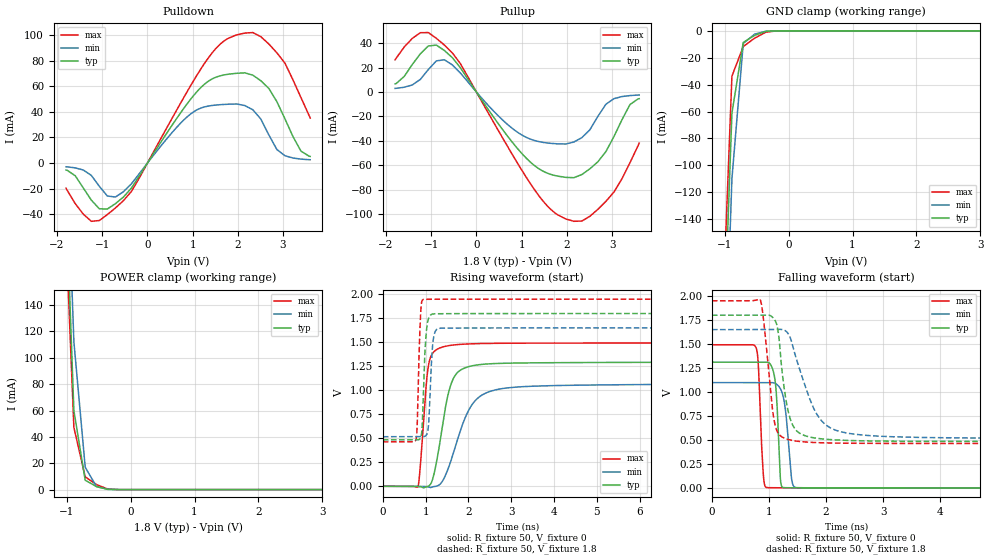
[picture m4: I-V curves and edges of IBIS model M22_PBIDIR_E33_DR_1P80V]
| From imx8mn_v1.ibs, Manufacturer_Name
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[Model] M22_PBIDIR_E33_DR_1P80V
Model_type I/O
Vinl  =  0.54
Vinh  =  1.26
Vmeas =  0.9
| Capacitance   typ   min   max
C_comp   8.99140471561e-13   8.21462742958e-13   9.40633374847e-13
| Variables   typ   min   max
[GND Clamp Reference]   0   0   0
[POWER Clamp Reference]   1.8   1.65   1.95
[Pulldown Reference]   0   0   0
[Pullup Reference]   1.8   1.65   1.95
[Temperature Range]   25   125   -40
[Voltage Range]   1.8   1.65   1.95
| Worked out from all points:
|   slope of the pulldown table from 0 to 0.27 V, typ, clamps not added: 18.2 ohm
|   slope of the pullup table from 0 to 0.27 V, typ, clamps not added: 18.3 ohm
|   GND clamp passes 1 mA (typ) near -0.39 V on its own axis
|   POWER clamp passes 1 mA (typ) near -0.43 V on its own axis
|   falling waveform, R_fixture 50, V_fixture 0: 20-80 % time 64.8ps typ, 101ps min, 63.2ps max; typ from 1.31 V to 0 V
|   falling waveform, R_fixture 50, V_fixture 1.8: 20-80 % time 178ps typ, 425ps min, 151ps max; typ from 1.8 V to 0.484 V
|   rising waveform, R_fixture 50, V_fixture 0: 20-80 % time 321ps typ, 562ps min, 154ps max; typ from 0 V to 1.3 V
|   rising waveform, R_fixture 50, V_fixture 1.8: 20-80 % time 72.2ps typ, 72.2ps min, 56.6ps max; typ from 0.484 V to 1.8 V
[GND Clamp]
| Voltage   I(typ)   I(min)   I(max)
-1.8V     -1.562A    -1.614A    -1.516A
-1.064V   -296mA     -355.2mA   -250.4mA
-886.4mV  -61.18mA   -109.9mA   -33.74mA
-709.1mV  -8.602mA   -9.384mA   -11.67mA
-531.8mV  -3.4mA     -2.481mA   -5.473mA
-354.5mV  -361.2uA   -272.6uA   -975.8uA
-177.3mV  -1.362uA   -3.436uA   -2.724uA
3.6V      0A         0A         0A
[POWER Clamp]
| Voltage   I(typ)   I(min)   I(max)
-1.8V     1.563A     1.607A     1.521A
-1.064V   296.1mA    350.6mA    257.7mA
-886.4mV  60.03mA    112.2mA    47.22mA
-709.1mV  7.094mA    16.96mA    9.663mA
-531.8mV  2.299mA    2.209mA    3.776mA
-354.5mV  136.5uA    326.9uA    430.1uA
-177.3mV  338.8nA    11.95uA    535.8nA
3.6V      0A         0A         0A
[Pulldown]
| Voltage   I(typ)   I(min)   I(max)
-1.8V     -5.447mA   -2.883mA   -19.62mA
-1.241V   -28.93mA   -9.601mA   -45.5mA
-1.064V   -35.72mA   -18.13mA   -44.9mA
-709.1mV  -31.73mA   -26.52mA   -35.12mA
-354.5mV  -19.54mA   -16.21mA   -22.17mA
956.3mV   49.91mA    38.39mA    60.51mA
1.519V    67.15mA    45.37mA    89.73mA
1.977V    70.19mA    46.16mA    100.2mA
2.332V    68.71mA    41.67mA    102mA
2.864V    48.01mA    10.59mA    86.16mA
3.395V    9.384mA    3.113mA    51.23mA
3.6V      5.213mA    2.619mA    35.18mA
[Pullup]
| Voltage   I(typ)   I(min)   I(max)
-1.8V     6.738mA    3.031mA    26.49mA
-1.241V   31.39mA    10.4mA     48.69mA
-886.4mV  38.53mA    25.6mA     44.07mA
-354.5mV  19.98mA    15.63mA    23.28mA
506.2mV   -27.09mA   -20.31mA   -32.95mA
1.097V    -54mA      -37.01mA   -69.56mA
1.575V    -66.58mA   -41.77mA   -93.63mA
1.977V    -69.95mA   -42.59mA   -104.1mA
2.509V    -62.92mA   -30.89mA   -101.8mA
2.864V    -48.77mA   -9.962mA   -89.63mA
3.395V    -10.24mA   -2.863mA   -57.98mA
3.6V      -5.395mA   -2.386mA   -41.8mA
[Ramp]
dV/dt_r   0.78173/0.320651n  0.652631/0.562174n  0.895239/0.153981n
dV/dt_f   0.789882/0.177801n  0.680105/0.424702n  0.892361/0.151285n
R_load = 50
[Falling Waveform]
R_fixture = 50
V_fixture = 0
V_fixture_min = 0
V_fixture_max = 0
| Time   V(typ)   V(min)   V(max)
0s        1.311V     1.098V     1.492V
772ps     1.311V     1.098V     1.464V
813.9ps   1.311V     1.098V     1.281V
916.2ps   1.311V     1.098V     53.5mV
1.117ns   1.071V     1.087V     1.095mV
1.219ns   21.9mV     1.011V     816.3uV
1.292ns   1.477mV    795.1mV    677.4uV
1.408ns   876.2uV    55.98mV    521.8uV
1.614ns   556.6uV    1.034mV    335.5uV
333.3ns   53.32nV    344.7nV    38.5nV
[Falling Waveform]
R_fixture = 50
V_fixture = 1.8
V_fixture_min = 1.65
V_fixture_max = 1.95
| Time   V(typ)   V(min)   V(max)
0s        1.8V       1.65V      1.95V
845.9ps   1.8V       1.65V      1.963V
909.8ps   1.8V       1.65V      1.731V
1.083ns   1.766V     1.651V     729.5mV
1.194ns   1.448V     1.653V     546.9mV
1.316ns   857.1mV    1.624V     508mV
1.466ns   607.4mV    1.373V     488.8mV
1.899ns   512.5mV    715.8mV    470.5mV
2.531ns   491.8mV    557.4mV    464.7mV
333.3ns   483.5mV    516.5mV    462.7mV
[Rising Waveform]
R_fixture = 50
V_fixture = 0
V_fixture_min = 0
V_fixture_max = 0
| Time   V(typ)   V(min)   V(max)
0s        34.82nV    339nV      30.15nV
822.2ps   -1.45mV    -3.956uV   -2.204mV
873.9ps   -4.915mV   26.44uV    198.9mV
1.036ns   -2.625mV   -5.03mV    1.159V
1.169ns   82.05mV    -5.771mV   1.389V
1.506ns   918.1mV    159.6mV    1.463V
1.678ns   1.147V     389.1mV    1.474V
2.089ns   1.256V     852.9mV    1.485V
2.638ns   1.279V     1.005V     1.49V
333.3ns   1.303V     1.088V     1.492V
[Rising Waveform]
R_fixture = 50
V_fixture = 1.8
V_fixture_min = 1.65
V_fixture_max = 1.95
| Time   V(typ)   V(min)   V(max)
0s        483.5mV    516.5mV    462.7mV
772.3ps   483.4mV    516.5mV    485.4mV
802.3ps   483mV      516.5mV    629.9mV
897.6ps   527.5mV    516.3mV    1.889V
1.007ns   1.564V     528.9mV    1.948V
1.067ns   1.748V     635.1mV    1.949V
1.107ns   1.781V     1.003V     1.949V
1.206ns   1.797V     1.591V     1.949V
1.589ns   1.799V     1.648V     1.95V
333.3ns   1.8V       1.65V      1.95V
[Add Submodel]
| Submodel Name Mode
M22_PBIDIR_E33_DR_1P80V_T All
